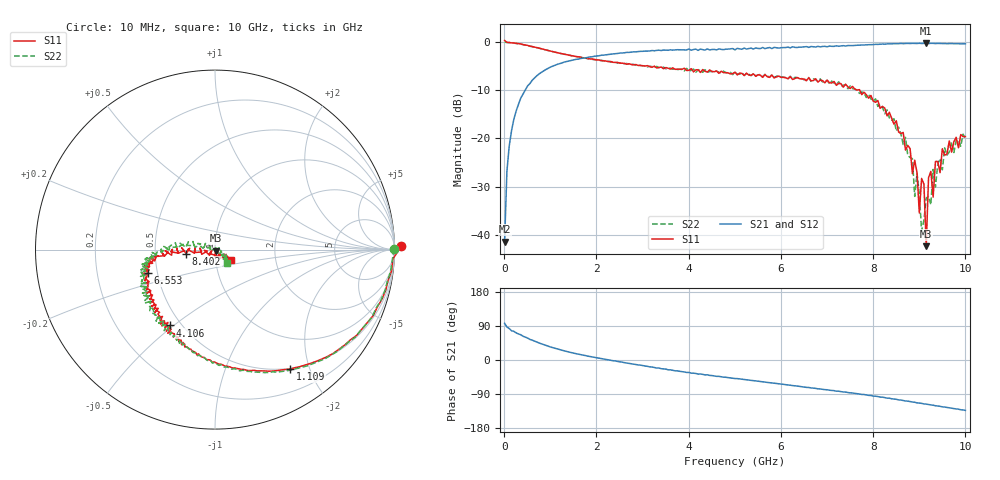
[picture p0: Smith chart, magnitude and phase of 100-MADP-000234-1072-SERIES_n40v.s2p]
!Agilent Technologies,E8364C,MY48140145,A.09.42.15
!Agilent E8364C: A.09.42.15
!Date: Wednesday, December 02, 2020 08:34:29
!Correction: S11(Full 2 Port(1,2))
!S21(Full 2 Port(1,2))
!S12(Full 2 Port(1,2))
!S22(Full 2 Port(1,2))
!S2P File: Measurements: S11, S21, S12, S22:
# Hz S  dB  R 50
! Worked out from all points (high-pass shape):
!   201 points, 10 MHz to 10 GHz, reference 50 ohm
!   highest |S21| = -0.26 dB at 9.151 GHz (marker M1); lowest = -41.4 dB at 10 MHz (marker M2)
!   |S21| within 3 dB of the highest: 1.781 GHz to end of sweep
!   lowest |S11| = -42.4 dB at 9.151 GHz (marker M3), VSWR 1.02, Z = 50.4 - j0.673 ohm
!   |S11| at or under -10 dB: 7.708 GHz to end of sweep
!   |S22| runs from -39.2 to 0.0 dB; largest |S21 - S12| = 0.021
!   S11 on the Smith chart (normalised r, x): 10 MHz: -41, +22; 1.109 GHz: 0.49, -1.70; 4.106 GHz: 0.44, -0.49; 6.553 GHz: 0.44, -0.14; 8.402 GHz: 0.72, -0.03; 10 GHz: 1.18, -0.14
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1e7  0.33 1.2  -41.42 96.8  -45.47 68.1  -0.02 0.2
5.995e7  -0.07 -3.2  -26.84 87.2  -26.88 85.9  -0.10 -4.0
2.098e8  -0.19 -13.3  -16.05 75.6  -16.06 75.1  -0.23 -13.8
1.1089e9  -2.09 -57.9  -4.78 30.4  -4.78 30.4  -2.12 -59.6
1.7083e9  -3.27 -76.5  -3.34 12.8  -3.32 13.0  -3.23 -78.4
3.35665e9  -5.26 -111.6  -1.70 -21.3  -1.69 -22.0  -5.35 -111.6
4.1059e9  -6.19 -120.5  -1.55 -34.8  -1.54 -34.6  -5.61 -124.3
5.005e9  -6.25 -133.6  -1.63 -49.0  -1.56 -48.3  -6.23 -142.5
6.55345e9  -8.05 -160.6  -0.95 -72.3  -0.94 -71.7  -7.76 -165.8
6.7033e9  -8.00 -163.3  -0.97 -74.3  -0.95 -73.9  -7.63 -168.0
8.35165e9  -14.59 176.9  -0.39 -100.8  -0.39 -101.5  -15.76 175.5
8.4016e9  -15.81 -172.2  -0.38 -102.3  -0.33 -101.7  -16.24 163.6
8.85115e9  -27.32 -169.6  -0.27 -110.8  -0.28 -110.5  -24.21 168.4
8.9011e9  -24.54 -175.8  -0.28 -111.5  -0.27 -112.0  -32.05 160.8
9.001e9  -35.50 -169.4  -0.26 -113.6  -0.28 -113.6  -31.53 -163.5
9.1009e9  -29.49 -79.3  -0.27 -115.9  -0.25 -115.2  -36.95 147.4
9.15085e9  -42.38 -61.4  -0.26 -116.4  -0.30 -116.8  -32.40 -55.4
9.2008e9  -28.16 -91.3  -0.32 -117.5  -0.25 -117.5  -32.04 23.5
9.3007e9  -32.18 -45.6  -0.27 -119.2  -0.27 -119.7  -26.44 -28.5
9.35065e9  -24.79 -58.5  -0.32 -120.7  -0.27 -120.2  -30.12 -7.0
9.55045e9  -23.49 -23.1  -0.31 -124.2  -0.32 -124.5  -21.97 -42.7
1e10  -19.63 -33.5  -0.36 -133.0  -0.36 -133.0  -20.04 -49.5
